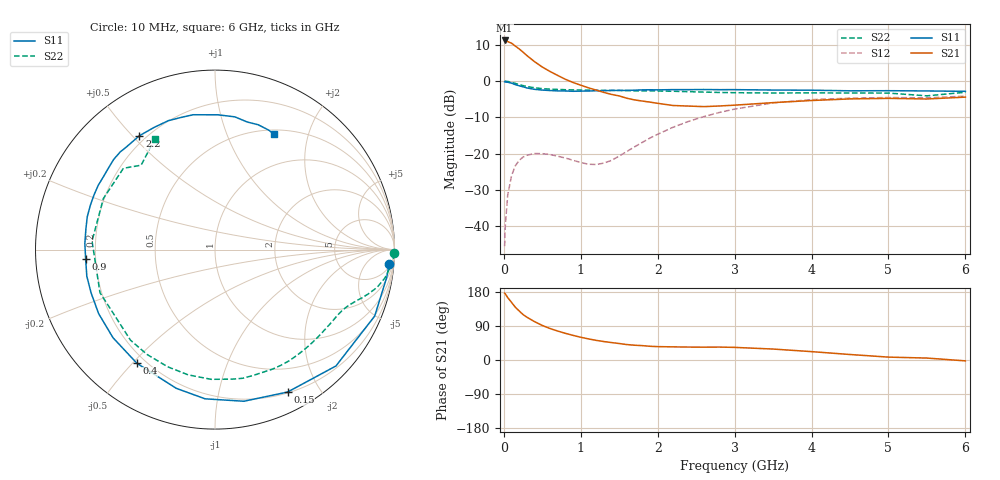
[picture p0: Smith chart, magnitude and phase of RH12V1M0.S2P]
! SIEMENS Small Signal Semiconductors
! BFR106
! Si NPN RF Bipolar Junction Transistor in SOT23
! VCE = 12 V  IC = 1 mA
! Common Emitter S-Parameters:  August  1996
# GHz  S  MA  R  50
!  f  S11  S21  S12  S22
! GHz  MAG  ANG  MAG  ANG  MAG  ANG  MAG  ANG
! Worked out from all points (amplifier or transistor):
!   36 points, 10 MHz to 6 GHz, reference 50 ohm
!   highest |S21| = 11.2 dB at 10 MHz (marker M1)
!   |S21| within 3 dB of that: start of sweep to 237.5 MHz
!   unconditionally stable (mu >= 1): 857.6 MHz to 1.826 GHz; 3.208 GHz to end of sweep
!   at 250 MHz: K = 0.25, MSG = 14.5 dB, |S12| = -21.0 dB
!   at 1.4 GHz: K = 1.40, MAG = 5.3 dB, |S12| = -21.9 dB
!   at 6 GHz: K = 1.02, MAG = -1.0 dB, |S12| = -4.2 dB
!   S11 on the Smith chart (normalised r, x): 10 MHz: 7, -22; 150 MHz: 0.21, -1.61; 400 MHz: 0.17, -0.51; 900 MHz: 0.16, -0.04; 2.2 GHz: 0.17, +0.52; 6 GHz: 0.56, +1.49
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0.01  0.9737 -4.7  3.624 176.3  0.0053 88.5  0.9999 -1.2
0.02  0.9691 -9.2  3.595 174.2  0.0106 84.2  0.997 -2.1
0.05  0.9638 -22.6  3.496 164.8  0.0266 77.1  0.9867 -5.0
0.1  0.9351 -43.9  3.322 152.1  0.0497 66.4  0.9597 -9.5
0.15  0.8907 -63.0  3.029 139.1  0.0681 55.4  0.9275 -13.1
0.2  0.8601 -79.2  2.767 129.3  0.0808 47.8  0.8946 -15.7
0.25  0.8332 -93.8  2.502 119.9  0.0896 40.7  0.8644 -18.0
0.3  0.8025 -105.6  2.243 112.9  0.095 36.0  0.8405 -19.7
0.4  0.7684 -124.5  1.847 101.1  0.1002 27.8  0.8072 -22.6
0.5  0.751 -139.2  1.559 91.1  0.0999 22.9  0.7864 -25.4
0.6  0.74 -151.2  1.355 83.1  0.0971 20.3  0.7736 -28.4
0.9  0.7226 -175.7  0.955 65.0  0.0809 22.9  0.755 -37.9
1.1  0.7284 170.8  0.807 55.7  0.0714 35.4  0.7489 -45.2
1.3  0.737 160.5  0.697 48.7  0.074 54.7  0.7451 -52.7
1.6  0.7426 146.7  0.579 40.7  0.1072 75.9  0.7385 -64.6
2.2  0.7615 123.6  0.46 34.7  0.2308 78.9  0.7231 -91.7
2.8  0.7602 104.4  0.453 34.1  0.3682 65.1  0.6962 -122.9
3.5  0.7512 88.8  0.504 28.9  0.4995 46.0  0.6842 -159.5
4.5  0.7333 75.8  0.567 14.5  0.5805 21.7  0.6839 155.4
5  0.736 70.9  0.577 7.6  0.5925 12.4  0.6823 138.4
5.5  0.7299 65.8  0.566 5.1  0.5868 7.9  0.6249 131.2
6  0.7214 62.8  0.6 -2.3  0.6194 -0.3  0.7007 118.7
